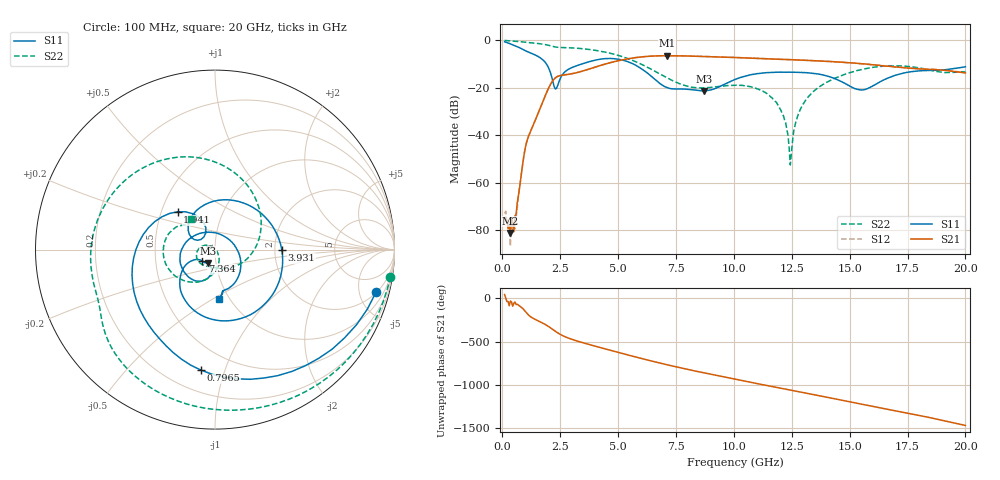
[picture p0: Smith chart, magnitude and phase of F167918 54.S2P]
!  2-Port S-parameters saved by WinCal
! VAR MeasName=S-Parameters (CALIBRATED_DATA) read from VNA (N5242A)
! VAR MeasDate=2016-11-22 10:27:27
! VAR NAME=F167918 54
! VAR FILENAME=F167918 54.S2P
! VAR DATE=2016-11-22 10:27:27
! VAR PHYS_PORTS=1,2
# Hz S DB R 50
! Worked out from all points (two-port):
!   401 points, 100 MHz to 20 GHz, reference 50 ohm
!   highest |S21| = -6.51 dB at 7.115 GHz (marker M1); lowest = -81.2 dB at 348.8 MHz (marker M2)
!   |S21| within 3 dB of the highest: 4.636 GHz to 15.01 GHz (10.37 GHz wide, 106 % of centre)
!   lowest |S11| = -21.3 dB at 8.707 GHz (marker M3), VSWR 1.19, Z = 45.7 - j7.03 ohm
!   |S11| at or under -10 dB: 1.904 GHz to 3.435 GHz (1.531 GHz wide, 57.3 % of centre); 5.656 GHz to end of sweep
!   |S22| runs from -52.5 to -0.1 dB; largest |S21 - S12| = 0.0044
!   S11 on the Smith chart (normalised r, x): 100 MHz: 2.08, -7.12; 796.5 MHz: 0.34, -0.83; 1.941 GHz: 0.61, +0.28; 3.931 GHz: 2.19, -0.01; 7.364 GHz: 0.86, -0.11; 20 GHz: 0.89, -0.53
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1e8  -0.65 -14.8  -74.83 43.1  -72.99 48.4  -0.10 -8.8
3.4875e8  -1.54 -46.3  -81.22 -31.7  -86.77 16.5  -0.26 -29.1
5.4775e8  -2.32 -69.1  -74.02 -42.8  -79.45 -95.1  -0.40 -44.8
7.965e8  -3.40 -96.6  -58.23 -98.2  -58.47 -96.3  -0.63 -63.5
1.095e9  -4.85 -126.5  -41.54 176.0  -41.49 176.6  -0.92 -84.5
1.94075e9  -10.56 134.7  -21.43 43.7  -21.41 43.7  -2.00 -136.6
2.33875e9  -20.31 144.1  -15.54 -30.0  -15.51 -29.9  -2.91 -154.6
3.43325e9  -10.01 48.0  -13.08 -150.0  -13.08 -149.9  -3.55 159.6
3.93075e9  -8.58 -0.3  -11.57 172.6  -11.56 172.8  -4.13 137.5
5.32375e9  -8.73 -105.4  -8.00 72.3  -7.96 72.2  -7.38 71.4
6.7665e9  -17.92 -153.7  -6.57 -25.9  -6.57 -26.1  -14.01 -9.1
7.11475e9  -19.94 -145.0  -6.51 -48.1  -6.53 -48.1  -15.87 -29.5
7.3635e9  -20.48 -137.8  -6.54 -63.5  -6.53 -63.6  -17.09 -44.2
8.70675e9  -21.33 -117.2  -6.82 -141.7  -6.81 -141.7  -20.05 -102.0
1.005e10  -16.55 -101.0  -7.26 144.7  -7.26 144.8  -18.98 -144.8
1.17415e10  -13.51 -131.1  -7.95 55.9  -7.90 55.8  -25.04 153.8
1.2438e10  -13.44 -144.1  -8.20 19.8  -8.17 19.4  -52.55 78.8
1.2836e10  -13.54 -152.3  -8.37 -1.1  -8.33 -1.4  -29.94 -56.1
1.338325e10  -13.94 -165.8  -8.58 -29.9  -8.56 -30.1  -22.14 -74.2
1.547275e10  -20.91 70.1  -9.87 -140.9  -9.92 -141.0  -12.43 -132.3
1.67165e10  -15.69 -28.6  -10.99 153.5  -11.02 154.0  -10.82 -169.2
2e10  -11.17 -85.5  -13.75 -29.1  -13.64 -29.2  -13.25 128.0
